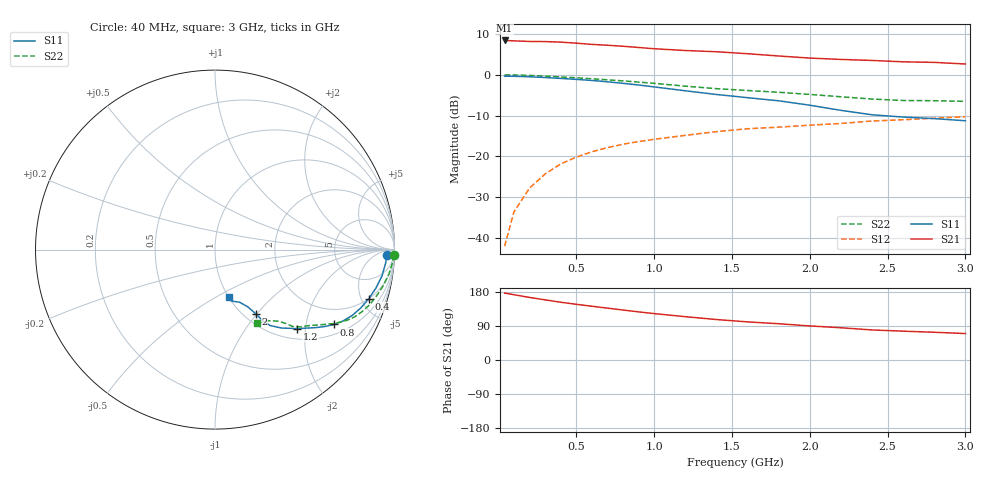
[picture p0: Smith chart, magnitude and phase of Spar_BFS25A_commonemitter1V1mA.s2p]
! Filename:  BFS25AD.S2P  Version:  4.0
! NXP part #: BFS25A  Date: Jun 1994
! Bias condition: Vce=1V, Ic=1mA
#  MHz  S  MA  R  50
! Freq  S11  S21  S12  S22  !GUM [dB]
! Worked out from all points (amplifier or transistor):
!   21 points, 40 MHz to 3 GHz, reference 50 ohm
!   highest |S21| = 8.4 dB at 40 MHz (marker M1)
!   |S21| within 3 dB of that: start of sweep to 1.5 GHz
!   unconditionally stable (mu >= 1): 1.972 GHz to end of sweep
!   at 300 MHz: K = 0.24, MSG = 16.2 dB, |S12| = -24.3 dB
!   at 1 GHz: K = 0.61, MSG = 11.1 dB, |S12| = -15.8 dB
!   at 3 GHz: K = 1.12, MAG = 4.3 dB, |S12| = -10.3 dB
!   lowest NFmin = 1.90 dB at 500 MHz
!   S11 on the Smith chart (normalised r, x): 40 MHz: 30, -22; 400 MHz: 1.99, -5.71; 800 MHz: 1.34, -2.90; 1.2 GHz: 1.22, -1.80; 2 GHz: 1.13, -0.98; 3 GHz: 1.01, -0.57
40  0.958 -1.8  2.617 176.6  0.008 89.4  0.995 -1.7
100  0.954 -4.4  2.587 172.3  0.021 84.6  0.992 -4.1
200  0.942 -8.9  2.545 165.1  0.041 80.9  0.978 -8.1
300  0.922 -13.4  2.535 158.7  0.061 77.5  0.959 -12.1
400  0.899 -17.8  2.497 152.5  0.081 74.6  0.937 -15.9
500  0.875 -21.8  2.425 147.0  0.098 71.8  0.915 -19.6
600  0.849 -25.5  2.344 141.9  0.114 69.2  0.89 -22.8
700  0.818 -29.0  2.288 136.9  0.128 67.2  0.865 -25.6
800  0.783 -32.2  2.223 131.9  0.141 65.3  0.839 -27.8
900  0.747 -35.0  2.148 127.0  0.152 63.2  0.811 -29.8
1000  0.708 -37.9  2.073 122.5  0.162 61.3  0.783 -31.7
1200  0.635 -43.9  1.972 114.3  0.181 57.7  0.723 -35.4
1400  0.572 -49.8  1.905 106.8  0.201 55.5  0.674 -38.9
1600  0.523 -54.0  1.802 100.6  0.218 53.3  0.64 -42.3
1800  0.479 -56.1  1.69 95.7  0.228 52.7  0.609 -44.7
2000  0.423 -57.6  1.594 89.9  0.241 51.5  0.573 -46.1
2200  0.366 -60.3  1.534 85.1  0.253 50.6  0.536 -48.2
2400  0.323 -65.1  1.491 79.3  0.271 49.1  0.503 -51.9
2600  0.303 -71.5  1.434 76.1  0.281 47.9  0.483 -56.2
2800  0.29 -74.4  1.412 73.2  0.293 48.4  0.48 -58.9
3000  0.273 -73.2  1.349 69.8  0.306 47.9  0.472 -60.1
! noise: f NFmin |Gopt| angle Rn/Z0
500  1.9  0.807  3  2.1
1000  2  0.814  10  2
2000  2.4  0.681  29  1.5
